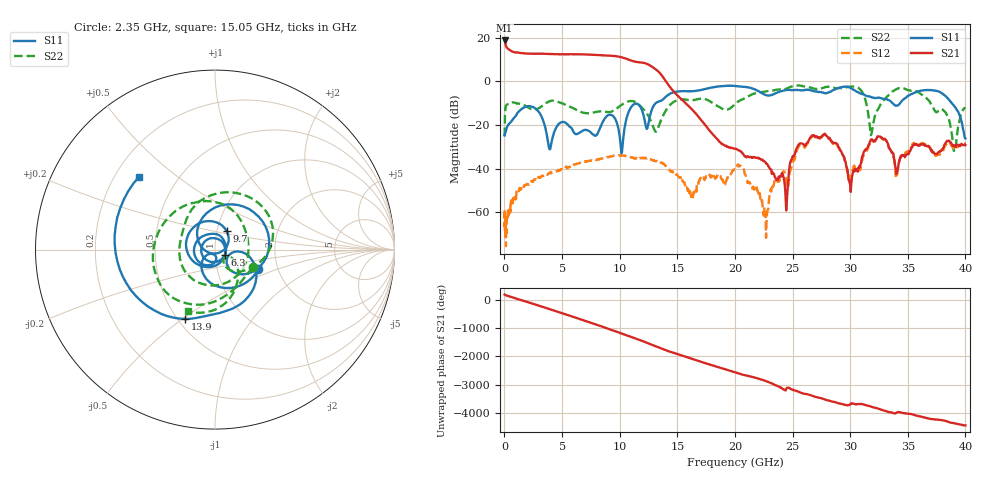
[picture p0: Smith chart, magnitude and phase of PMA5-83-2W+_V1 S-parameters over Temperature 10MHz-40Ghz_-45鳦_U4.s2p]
!Mini-Circuits Laboratory
!S-Parameters
!Model: US-AMP-1
!Run / Lot / Date Code: N/A / N/A / N/A
!Fixture: N/A, Pressing Arm: N/A
!Network Analyzer: NFA N8975A;  Serial number: 74408
!Date: 11/29/2023 at 10:17:41 AM
!No.: Unit# 1 (U4)
!Tested with: -45°C
! 2 port cal with Bias Tee PE1622 in line. No normalization applied. Bias cond 2: Vdd= 12V, Idd= 400mA, Vg2= 5V, starting point for Vg1= -2V
# Hz  S  dB  R  50
!Frequency  S11 dB  S11 Deg  S21 dB  S21 Deg  S12 dB  S12 Deg  S22 dB  S22 Deg
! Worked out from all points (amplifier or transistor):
!   826 points, 10 MHz to 40 GHz, reference 50 ohm
!   highest |S21| = 18.8 dB at 10 MHz (marker M1)
!   |S21| within 3 dB of that: start of sweep to 167.6 MHz
!   unconditionally stable (mu >= 1): start of sweep to end of sweep
!   at 5.6 GHz: K = 10.01, MAG = 12.8 dB, |S12| = -39.2 dB
!   at 19.4 GHz: K = 860.12, MAG = -25.4 dB, |S12| = -44.0 dB
!   at 40 GHz: K = 363.63, MAG = -28.9 dB, |S12| = -28.6 dB
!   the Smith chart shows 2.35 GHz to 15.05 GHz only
!   S11 on the Smith chart (normalised r, x): 2.35 GHz: 1.58, -0.37; 6.3 GHz: 1.11, -0.06; 9.7 GHz: 1.11, +0.23; 13.9 GHz: 0.55, -0.51; 15.05 GHz: 0.30, +0.37
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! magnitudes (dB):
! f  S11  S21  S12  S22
! 10 MHz  -24.7  18.8  -59.1  -25.1
! 2.35 GHz  -11.5  12.7  -45.7  -12.7
! 3.9 GHz  -31.0  12.6  -42.1  -9.1
! 6.3 GHz  -24.1  12.5  -37.8  -13.1
! 6.7 GHz  -22.9  12.4  -37.3  -14.1
! 9.7 GHz  -18.3  11.5  -34.1  -12.6
! 10.15 GHz  -33.0  11.1  -34.0  -10.8
! 11.1 GHz  -11.1  9.4  -34.8  -9.0
! 13.35 GHz  -9.3  4.5  -36.8  -21.1
! 13.9 GHz  -7.5  0.9  -38.1  -14.3
! 15.05 GHz  -4.6  -6.6  -43.4  -8.5
! 20.05 GHz  -2.1  -31.0  -40.5  -10.2
! 22.65 GHz  -6.2  -37.1  -60.4  -4.6
! 24.45 GHz  -3.9  -59.2  -45.2  -3.4
! 26.7 GHz  -4.2  -24.8  -25.3  -3.0
! 30 GHz  -2.9  -47.3  -47.7  -2.4
! 31.85 GHz  -7.3  -26.7  -26.9  -24.0
! 33.35 GHz  -8.6  -30.4  -30.1  -6.2
! 34.05 GHz  -11.1  -41.8  -43.8  -3.5
! 38.1 GHz  -6.0  -30.4  -31.4  -13.3
! 39.05 GHz  -11.4  -29.4  -30.6  -31.0
! 40 GHz  -26.1  -29.2  -28.6  -12.5
